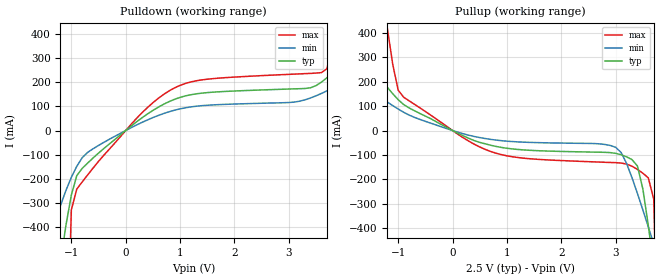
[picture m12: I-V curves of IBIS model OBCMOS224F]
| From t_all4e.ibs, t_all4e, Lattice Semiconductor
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|   OBCMOS224F
[Model]   OBCMOS224F
Model_type   Output
Polarity   Non-Inverting
C_comp   2pF   2pF   2pF
[Temperature Range]   25.0000   125.0000   -40.0000
[Voltage Range]   2.5000V   2.3000V   2.7000V
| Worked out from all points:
|   slope of the pulldown table from 0 to 0.375 V, typ, clamps not added: 5.83 ohm
|   slope of the pullup table from 0 to 0.375 V, typ, clamps not added: 9.61 ohm
[Pulldown]
|voltage   I(typ)   I(min)   I(max)
-2.5V     -2.953A    -1.245A    -25.87A
-1.4V     -892.1mA   -445.3mA   -5.973A
-1.1V     -392.3mA   -247.7mA   -1.134A
-900mV    -186.4mA   -147.6mA   -241.7mA
-800mV    -156.1mA   -112.2mA   -212mA
300mV     52.54mA    33.62mA    73.23mA
900mV     128.9mA    83.99mA    176mA
3.4V      176.4mA    134.4mA    235.7mA
3.7V      217.6mA    163.7mA    254.8mA
3.9V      261mA      188.5mA    485.4mA
4.5V      422.4mA    281.3mA    1.466A
5V        578.9mA    371.2mA    2.341A
[Pullup]
|voltage   I(typ)   I(min)   I(max)
-2.5V     568.3mA    341.1mA    2.668A
-2V       409.8mA    248.2mA    1.78A
-1.2V     176.7mA    116.3mA    418.3mA
-1V       126mA      87.81mA    164.7mA
400mV     -41.34mA   -24.39mA   -56.12mA
1.2V      -77.41mA   -46.41mA   -110.3mA
3V        -93.31mA   -68.52mA   -131.4mA
3.4V      -145mA     -257.3mA   -158.7mA
3.6V      -388.3mA   -394mA     -193.5mA
3.7V      -556.4mA   -464.4mA   -280.5mA
3.8V      -732.4mA   -535.6mA   -1.117A
5V        -2.977A    -1.415A    -22.23A
[Ramp]
| variable   typ   min   max
dV/dt_r   1.2302/0.2319ns   0.9845/0.4297ns   1.4301/0.1214ns
dV/dt_f   1.3495/0.2982ns   1.1782/0.7105ns   1.4950/0.1354ns
